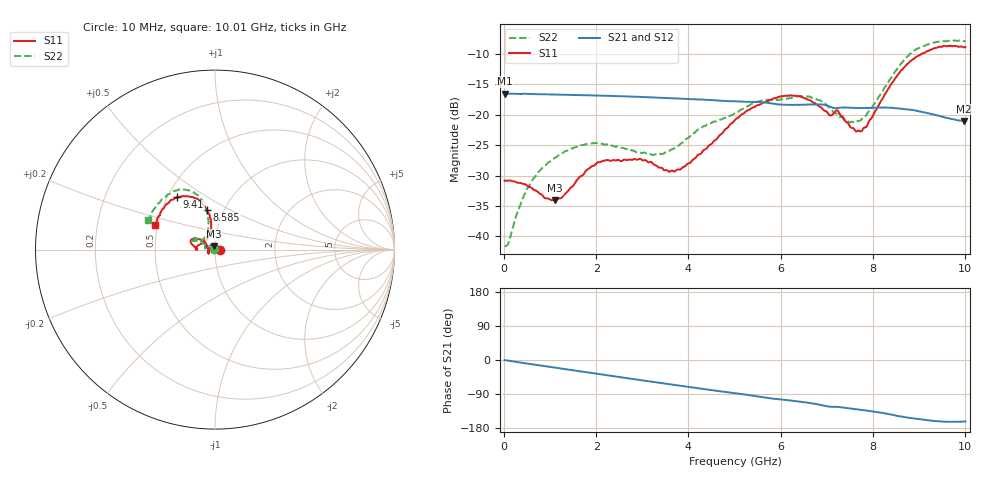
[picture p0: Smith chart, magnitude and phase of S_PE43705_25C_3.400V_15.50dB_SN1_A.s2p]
! Device ID: PE43705
! Serial: 1
! Insertion: A
! Impedance: 50 ohm
! Temp: 25C
! VDD: 3.400V
! Attenuation Step: 15.50dB
#  Hz  S  RI  R  50
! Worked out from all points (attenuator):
!   401 points, 10 MHz to 10.01 GHz, reference 50 ohm
!   highest |S21| = -16.50 dB at 10 MHz (marker M1); lowest = -21.0 dB at 9.985 GHz (marker M2)
!   lowest |S11| = -34.1 dB at 1.11 GHz (marker M3), VSWR 1.04, Z = 49.3 + j1.84 ohm
!   |S11| at or under -10 dB: start of sweep to 9.056 GHz
!   |S22| runs from -41.6 to -7.8 dB; largest |S21 - S12| = 0.0015
!   S11 on the Smith chart (normalised r, x): 10 MHz: 1.06, +0.00; 8.585 GHz: 0.84, +0.38; 9.41 GHz: 0.56, +0.38; 10.01 GHz: 0.48, +0.15
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1e7  0.0287 0.000252  0.1496 -0.000602  0.1496 -0.00065  -0.00832 0.00057
1.1e8  0.0286 0.00346  0.149 -0.00557  0.149 -0.00548  -0.00756 0.0052
5.35e8  0.0193 0.0169  0.146 -0.0258  0.1461 -0.0257  -0.014 0.0217
1.11e9  -0.00651 0.0186  0.1375 -0.0508  0.1376 -0.0507  -0.0345 0.028
1.685e9  -0.031 0.00503  0.125 -0.0736  0.125 -0.0736  -0.0523 0.0209
2.21e9  -0.0405 -0.0124  0.1102 -0.0918  0.1102 -0.0917  -0.0562 0.0102
2.96e9  -0.0376 -0.0216  0.0842 -0.1123  0.0844 -0.1122  -0.0478 0.00956
3.36e9  -0.033 -0.0162  0.069 -0.1197  0.0694 -0.1196  -0.0453 0.0124
3.86e9  -0.0363 0.00389  0.0496 -0.1264  0.0498 -0.1262  -0.0535 0.0245
5.01e9  -0.0734 0.0535  0.00515 -0.1289  0.00537 -0.129  -0.0885 0.054
5.985e9  -0.1291 0.0576  -0.0291 -0.1181  -0.0285 -0.118  -0.1182 0.0611
6.685e9  -0.1253 0.0256  -0.0508 -0.1105  -0.0506 -0.1106  -0.1281 0.051
7.06e9  -0.0989 0.00592  -0.064 -0.0978  -0.0638 -0.0981  -0.1028 0.0503
7.235e9  -0.108 0.0111  -0.0634 -0.0949  -0.0631 -0.0949  -0.0879 0.0482
7.435e9  -0.0813 0.0303  -0.0688 -0.0916  -0.0686 -0.0918  -0.0709 0.0562
7.71e9  -0.0507 0.0534  -0.075 -0.0857  -0.0744 -0.086  -0.0525 0.0722
8.36e9  -0.0236 0.1677  -0.0916 -0.0686  -0.0911 -0.069  -0.041 0.1886
8.585e9  -0.0437 0.2185  -0.0955 -0.0588  -0.0949 -0.0596  -0.0599 0.2485
8.935e9  -0.0963 0.2827  -0.0981 -0.0456  -0.0978 -0.045  -0.1236 0.3219
9.41e9  -0.2107 0.2917  -0.0937 -0.0312  -0.0934 -0.0308  -0.2319 0.3258
9.985e9  -0.3259 0.1481  -0.0849 -0.0271  -0.0849 -0.0272  -0.3632 0.1763
1.001e10  -0.3335 0.1392  -0.0855 -0.0271  -0.0852 -0.0274  -0.3713 0.1656
